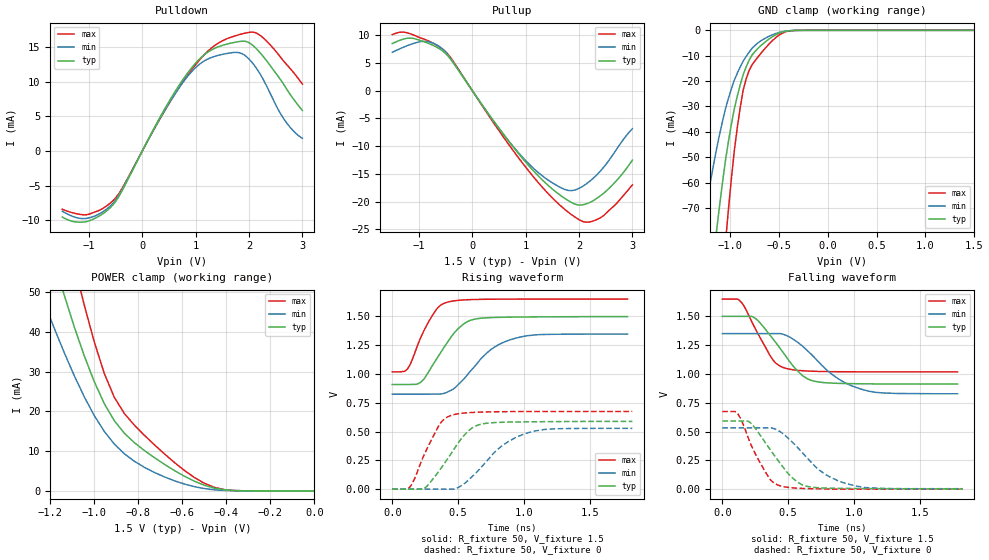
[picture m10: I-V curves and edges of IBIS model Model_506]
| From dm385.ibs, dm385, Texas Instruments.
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| Model based on original model for BCSHTLTCSCDDVPBFZ_SSDHV
|   Sub model SR01_5MA_PADN_10PER_1P5
[model]   Model_506
|[Description]  [1.5V-3-STATE-NOTERM-FAST:5MA, IND, 10%]
|   Fast slew rate (SR[1:0] = "10"), 1.60 * RExt = 0.625 * Iout
|   (I[2:0] = "000"), 5mA nominal with Rext = 50R,ODT off (ODT[1:0]
|   = "00") CMOS mode,Industrial temperature range (-40C to 125C,
|   25C nominal),10% power supply tolerance
|[Input Load]   NOTERM
|[Output Drive] FAST:5MA
|Voltage   1.5V
|Mode   3-STATE
Model_type   3-state
Polarity   Non-Inverting
Enable   Active-Low
Cref =  15pF
Rref =  100.0000M
Vref =  0V
Vmeas =  0.75
C_comp   1.865048p   1.676829p   1.989968p
[Temperature Range]   25   125   -40
[Voltage Range]   1.5   1.35   1.65
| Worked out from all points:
|   slope of the pulldown table from 0 to 0.225 V, typ, clamps not added: 67.2 ohm
|   slope of the pullup table from 0 to 0.225 V, typ, clamps not added: 72 ohm
|   GND clamp passes 1 mA (typ) near -0.49 V on its own axis
|   POWER clamp passes 1 mA (typ) near -0.47 V on its own axis
|   rising waveform, R_fixture 50, V_fixture 1.5: 20-80 % time 209ps typ, 270ps min, 155ps max; typ from 0.908 V to 1.5 V
|   rising waveform, R_fixture 50, V_fixture 0: 20-80 % time 219ps typ, 293ps min, 163ps max; typ from 0 V to 0.588 V
|   falling waveform, R_fixture 50, V_fixture 1.5: 20-80 % time 238ps typ, 314ps min, 176ps max; typ from 1.5 V to 0.912 V
|   falling waveform, R_fixture 50, V_fixture 0: 20-80 % time 228ps typ, 297ps min, 169ps max; typ from 0.591 V to 0.002 V
[POWER_clamp]
-1.5V     126mA      88.79mA    168.7mA
-1.242V   69.8mA     49.45mA    94.34mA
-1.136V   49.16mA    34.72mA    67.51mA
-1.061V   36.35mA    25.4mA     50.03mA
-1.045V   33.92mA    23.63mA    46.66mA
-954.5mV  21.93mA    14.95mA    29.5mA
-909.1mV  17.64mA    11.79mA    23.52mA
-863.6mV  14.51mA    9.351mA    19.47mA
-772.7mV  10.16mA    5.94mA     13.99mA
-590.9mV  3.705mA    1.741mA    5.166mA
-454.5mV  710.5uA    279.1uA    892.1uA
0V        1.424nA    14.34nA    3.127nA
[Pulldown]
-1.5V     -9.559mA   -8.721mA   -8.435mA
-1V       -10.13mA   -9.69mA    -9.153mA
-727.3mV  -9.021mA   -8.741mA   -8.25mA
-500mV    -7.306mA   -7.092mA   -6.791mA
272.7mV   4.034mA    3.899mA    3.845mA
681.8mV   9.399mA    9.044mA    9.061mA
1.045V    13.08mA    12.37mA    12.91mA
1.364V    14.86mA    13.69mA    15.28mA
1.818V    15.82mA    14.2mA     16.81mA
2.136V    14.79mA    11.98mA    17.05mA
2.636V    9.781mA    4.81mA     13.11mA
3V        5.846mA    1.81mA     9.659mA
[Pullup]
-1.5V     8.494mA    6.914mA    10.1mA
-1.273V   9.331mA    7.894mA    10.52mA
-954.5mV  8.972mA    8.846mA    9.444mA
-590.9mV  7.379mA    7.751mA    7.725mA
-409.1mV  5.694mA    5.824mA    5.984mA
909.1mV   -11.84mA   -11.65mA   -12.64mA
1.318V    -16.14mA   -15.4mA    -17.46mA
1.773V    -19.65mA   -17.92mA   -21.7mA
2.045V    -20.6mA    -17.37mA   -23.48mA
2.318V    -19.49mA   -15.31mA   -23.28mA
2.682V    -16.43mA   -10.88mA   -20.53mA
3V        -12.52mA   -6.85mA    -16.98mA
[GND_clamp]
-1.5V     -219.3mA   -131.6mA   -364.3mA
-1.288V   -134.4mA   -79.74mA   -225.6mA
-1.258V   -122.9mA   -72.77mA   -206.3mA
-1.136V   -79.27mA   -46.88mA   -132.4mA
-1.045V   -51.5mA    -31.06mA   -84.11mA
-1.015V   -44.02mA   -26.9mA    -70.91mA
-954.5mV  -31.01mA   -19.7mA    -47.55mA
-863.6mV  -17.48mA   -12.16mA   -23.55mA
-803mV    -11.81mA   -8.597mA   -15.85mA
-681.8mV  -5.986mA   -4.096mA   -9.026mA
-378.8mV  -126.2uA   -131.8uA   -179.7uA
1.5V      1.424nA    207.1nA    1.498nA
[Ramp]
dV/dt_f 0.35636293/0.24122199n 0.31607389/0.31711512n 0.38023247/0.17645022n
dV/dt_r 0.35610801/0.22162741n 0.31973955/0.29600616n  0.4054995/0.16321522n
R_load = 50
[Rising Waveform]
R_fixture = 50
V_fixture = 1.5
V_fixture_min = 1.35
V_fixture_max = 1.65
0s        908.2mV    824.1mV    1.018V
115.8ps   908.2mV    824.1mV    1.044V
221.1ps   933.1mV    824.1mV    1.329V
335.6ps   1.129V     825.3mV    1.561V
415ps     1.268V     841mV      1.622V
578.2ps   1.458V     1.004V     1.645V
742.1ps   1.489V     1.206V     1.649V
885.9ps   1.493V     1.293V     1.65V
1.09ns    1.495V     1.34V      1.65V
1.787ns   1.498V     1.347V     1.65V
[Rising Waveform]
R_fixture = 50
V_fixture = 0
V_fixture_min = 0
V_fixture_max = 0
0s        0V         0V         0V
130.9ps   0V         0V         15.29mV
256.5ps   18.6mV     0V         333.7mV
363.1ps   170mV      0V         568mV
456ps     325.4mV    0V         643.4mV
554ps     477.6mV    54.18mV    661.6mV
634.2ps   549mV      138.9mV    667.2mV
834.8ps   580.7mV    377.8mV    672.5mV
1.014ns   584.4mV    483.2mV    673.8mV
1.823ns   587.9mV    527.8mV    674.5mV
[Falling Waveform]
R_fixture = 50
V_fixture = 1.5
V_fixture_min = 1.35
V_fixture_max = 1.65
0s        1.499V     1.349V     1.649V
127.7ps   1.499V     1.349V     1.64V
237.7ps   1.491V     1.349V     1.421V
379.9ps   1.311V     1.349V     1.128V
471.9ps   1.171V     1.34V      1.052V
583.9ps   1.012V     1.264V     1.029V
662.6ps   949.4mV    1.184V     1.024V
854.1ps   918.9mV    978.6mV    1.019V
1.051ns   914.2mV    868.6mV    1.018V
1.787ns   911.5mV    827.6mV    1.017V
[Falling Waveform]
R_fixture = 50
V_fixture = 0
V_fixture_min = 0
V_fixture_max = 0
0s        591.1mV    531.7mV    673.5mV
110.8ps   591.1mV    531.7mV    663.8mV
211.6ps   578mV      531.7mV    403.6mV
352.6ps   361.5mV    531.7mV    102.8mV
431.5ps   235.9mV    504.4mV    32.05mV
614.2ps   34.46mV    308.9mV    6.325mV
767.5ps   10.26mV    139.8mV    2.493mV
919ps     6.66mV     56.49mV    0V
1.081ns   5.186mV    13.89mV    0V
1.823ns   2.423mV    4.066mV    0V
